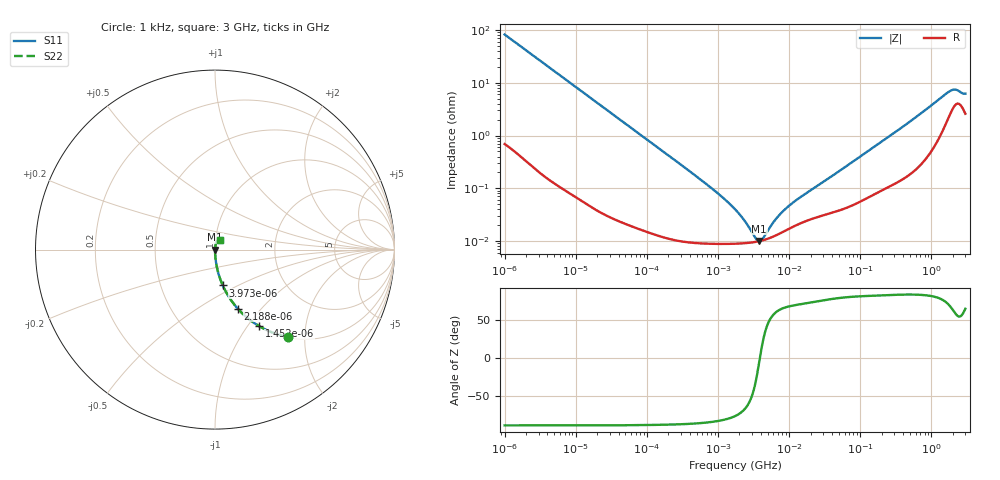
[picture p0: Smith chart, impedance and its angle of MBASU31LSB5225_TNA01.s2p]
! MBASU31LSB5225_TNA01  S-PARAMETER MODEL  ( Standard Model )
! Model Generated by TAIYO YUDEN Corporation (http://www.ty-top.com)
! Version 1.0
! TAIYO YUDEN Control No. 220601
! Copyright(c) 2012 TAIYO YUDEN CO.,LTD. All Rights Reserved.
! Product Description (link to TY-COMPAS)
! https://ds.yuden.co.jp/TYCOMPAS/or/detail?pn=MBASU31LSB5225KTNA01&u=M
! Products Name : Multilayer Ceramic Capacitors
! Characteristics :
!  Capacitance : 2.2 [uF] , Rated Voltage : 50 [V] , TCC : X5R
!  Case Size : 3.2 x 1.6 / 0.126 x 0.063 [mm/inch] , Thickness : 1.6 / 0.063 [mm/inch]
!  (Conditions: Temperature = 25 [degC] , DC Bias Voltage = 0 [V])
! External Node Assignments :
!  1  o---| |---o  2
! GND o---------o GND
! Frequency Range : 1kHz  -  3GHz  [ 401 STEP ]
# MHZ S RI R 50
! Freq[MHz].  S11 Real  S11 Imag  S21 Real  S21 Imag  S12 Real  S12 Imag  S22 Real  S22 Imag
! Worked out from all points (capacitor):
!   401 points, 1 kHz to 3 GHz, reference 50 ohm
!   read as one part in series: C = 1.93 uF near 1.077 kHz
!   lowest |Z| = 9.99 mohm at 3.79 MHz (marker M1)
!   series resonance near 3.876 MHz, so ESL is about 870 pH
!   S11 on the Smith chart (normalised r, x): 1 kHz: 1.01, -1.65; 1.452 kHz: 1.01, -1.14; 2.188 kHz: 1.01, -0.76; 3.973 kHz: 1.00, -0.42; 3 GHz: 1.05, +0.11
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0.001  0.4049 -0.4867  0.5951 0.4867  0.5951 0.4867  0.4049 -0.4867
0.001452  0.2461 -0.4266  0.7539 0.4266  0.7539 0.4266  0.2461 -0.4266
0.002188  0.127 -0.3292  0.873 0.3292  0.873 0.3292  0.127 -0.3292
0.003973  0.0431 -0.1995  0.9569 0.1995  0.9569 0.1995  0.0431 -0.1995
0.006696  0.0161 -0.122  0.9839 0.122  0.9839 0.122  0.0161 -0.122
0.01216  0.00524 -0.0681  0.9948 0.0681  0.9948 0.0681  0.00524 -0.0681
0.033275  0.000897 -0.0251  0.9991 0.0251  0.9991 0.0251  0.000897 -0.0251
0.147855  0.000157 -0.0057  0.9998 0.0057  0.9998 0.0057  0.000157 -0.0057
0.791611  8.97e-05 -0.00103  0.9999 0.00103  0.9999 0.00103  8.97e-05 -0.00103
1.732051  8.91e-05 -0.000392  0.9999 0.000392  0.9999 0.000392  8.91e-05 -0.000392
2.334012  9.09e-05 -0.000231  0.9999 0.000231  0.9999 0.000231  9.09e-05 -0.000231
3.388684  9.65e-05 -5.86e-05  0.9999 5.86e-05  0.9999 5.86e-05  9.65e-05 -5.86e-05
3.789741  9.94e-05 -9.66e-06  0.9999 9.66e-06  0.9999 9.66e-06  9.94e-05 -9.66e-06
4.238263  0.000103 3.88e-05  0.9999 -3.88e-05  0.9999 -3.88e-05  0.000103 3.88e-05
6.153411  0.000124 0.000203  0.9999 -0.000203  0.9999 -0.000203  0.000124 0.000203
8.291982  0.00015 0.000342  0.9998 -0.000342  0.9998 -0.000342  0.00015 0.000342
12.03889  0.000194 0.000537  0.9998 -0.000537  0.9998 -0.000537  0.000194 0.000537
21.06097  0.000264 0.000922  0.9997 -0.000922  0.9997 -0.000922  0.000264 0.000922
256.0921  0.00117 0.00957  0.9988 -0.00957  0.9988 -0.00957  0.00117 0.00957
1780.008  0.0267 0.0611  0.9733 -0.0611  0.9733 -0.0611  0.0267 0.0611
2144.796  0.0398 0.0596  0.9602 -0.0596  0.9602 -0.0596  0.0398 0.0596
3000  0.0282 0.0536  0.9718 -0.0536  0.9718 -0.0536  0.0282 0.0536
